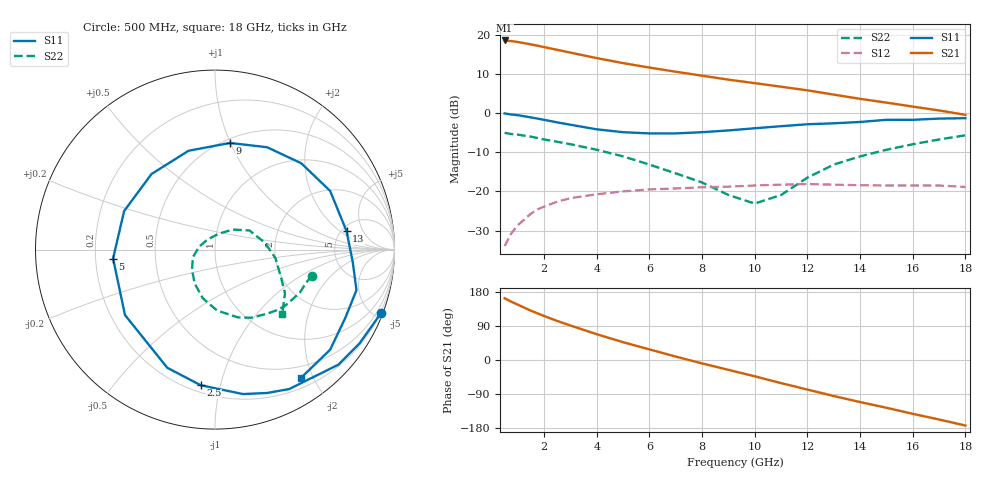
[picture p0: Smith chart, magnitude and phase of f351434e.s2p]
!ATF-35143
!S-PARAMETERS at Vds=4V  Id=30mA.  LAST UPDATED 06-3-99
# ghz s ma r 50
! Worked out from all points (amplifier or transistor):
!   23 points, 500 MHz to 18 GHz, reference 50 ohm
!   highest |S21| = 18.5 dB at 500 MHz (marker M1)
!   |S21| within 3 dB of that: start of sweep to 2.925 GHz
!   unconditionally stable (mu >= 1): 6.874 GHz to end of sweep
!   at 1.5 GHz: K = 0.30, MSG = 21.6 dB, |S12| = -25.7 dB
!   at 7 GHz: K = 1.01, MAG = 14.2 dB, |S12| = -19.3 dB
!   at 18 GHz: K = 1.31, MAG = 5.9 dB, |S12| = -18.9 dB
!   lowest NFmin = 0.10 dB at 500 MHz
!   S11 on the Smith chart (normalised r, x): 500 MHz: 0.15, -5.39; 2.5 GHz: 0.24, -0.87; 5 GHz: 0.27, -0.04; 9 GHz: 0.54, +1.00; 13 GHz: 5.52, +2.51; 18 GHz: 0.33, -1.83
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0.5  0.99 -21.0  8.45 163.0  0.02 78.0  0.56 -15.0
0.75  0.96 -33.0  8.3 154.0  0.029 70.0  0.54 -20.0
1  0.94 -43.0  8.07 146.0  0.037 65.0  0.53 -27.0
1.5  0.88 -62.0  7.53 130.0  0.052 54.0  0.5 -39.0
1.75  0.85 -70.0  7.24 123.0  0.059 49.0  0.48 -45.0
2  0.82 -79.0  6.95 116.0  0.064 45.0  0.46 -51.0
2.5  0.76 -96.0  6.41 103.0  0.074 36.0  0.43 -62.0
3  0.71 -112.0  5.91 91.0  0.082 28.0  0.4 -71.0
4  0.62 -144.0  5.03 68.0  0.092 14.0  0.34 -88.0
5  0.57 -175.0  4.34 47.0  0.1 1.0  0.28 -104.0
6  0.55 157.0  3.81 28.0  0.106 -11.0  0.22 -121.0
7  0.55 130.0  3.37 9.0  0.109 -23.0  0.17 -139.0
8  0.57 105.0  3 -9.0  0.113 -33.0  0.13 -161.0
9  0.6 82.0  2.67 -26.0  0.115 -44.0  0.09 170.0
10  0.64 63.0  2.41 -43.0  0.119 -54.0  0.07 129.0
11  0.68 45.0  2.17 -61.0  0.122 -66.0  0.09 78.0
12  0.72 27.0  1.95 -78.0  0.124 -77.0  0.15 48.0
13  0.74 8.0  1.72 -95.0  0.122 -89.0  0.22 29.0
14  0.77 -5.0  1.52 -111.0  0.12 -98.0  0.28 8.0
15  0.82 -16.0  1.36 -126.0  0.119 -108.0  0.34 -8.0
16  0.82 -28.0  1.21 -142.0  0.119 -118.0  0.4 -23.0
18  0.86 -56.0  0.95 -173.0  0.114 -140.0  0.52 -44.0
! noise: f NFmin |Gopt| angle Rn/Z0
0.5  0.1  0.9  4  0.22
0.9  0.14  0.85  13  0.21
1.5  0.21  0.77  26  0.18
1.8  0.25  0.73  33  0.17
2.5  0.33  0.64  49  0.15
3  0.38  0.58  62  0.14
5  0.62  0.4  121  0.07
6  0.74  0.35  154  0.05
8  0.99  0.31  -138  0.09
10  1.24  0.39  -72  0.26
